(* Logix 5000 AddOnInstructionDefinition export CM1T_DataExchange; software revision 20.00 *)

TYPE CM1T_DriveStatus :
STRUCT
   StatusValue : SINT;   // Indicates status and error type
   StatusValue1 : SINT;   // Additional status values
   In_Position : BOOL;   // Drive is in position and ready to move
   Moving : BOOL;   // Drive is currently moving
   Disabled : BOOL;   // Drive is disabled
   Error : BOOL;   // Drive is in an error state
   MoveComplete : BOOL;   // Move Complete
   NewStartRequired : BOOL;   // New setpoint required
   HomeAchieved : BOOL;   // Home achieved
END_STRUCT
END_TYPE

TYPE CM1T_Controlword :
STRUCT
   Start : BOOL;   // Start a motion or set a new setpoint
   Halt : BOOL;   // Halt the current motion
   Relative_Move : BOOL;   // Execute the position profile as a relative move
   Speed_Control : BOOL;   // Execute the profile as speed control only
   Disable : BOOL;   // Disable the drive (zero torque)
   Reset_Error : BOOL;   // Reset any existing errors with rising edge
   Set_to_Zero : BOOL;   // Set the current position to 0
   Home : BOOL;   // Execute a home search
END_STRUCT
END_TYPE

TYPE CM1T_Axis :
STRUCT
   Input : SINT[36];   // Data coming from the CM1-T
   Output : SINT[28];   // Data going to the CM1-T
   us50Counter : DINT;   // Controller 50us counter
   ModeOfOperation : SINT;   // Type of motion control mode
   ModeOfOperationDisplay : SINT;   // Indicates the active control mode
   Controlword : CM1T_Controlword;   // Controls the drive operation
   DriveStatus : CM1T_DriveStatus;   // Shows status of the drive
   PositionTarget : DINT;   // Final target position for position move
   SpeedTarget : DINT;   // Maximum speed for target move
   TorqueTarget : INT;   // Max torque allowed in 0.1% of peak. Typically 1100
   AccelerationTarget : INT;   // Acceleration for profile move
   DecelerationTarget : INT;   // Deceleration for profile move
   PositionActual : DINT;   // Actual position of the drive
   TargetActual : DINT;   // 1ms position target
   PositionError : DINT;   // Error between the current drive position and the instantaneous target position
   SpeedActual : DINT;   // Actual speed of the drive
   CurrentActual : INT;   // 0.1% of rated current
   OverloadActual : INT;   // 0.1% of overload torque
   DCVoltage : INT;   // DC voltage bus. 0.1V unit
   AnalogIN : INT;   // Value of 10bit analog input
   DigitalIN : SINT;   // Read the digital inputs
   DigitalOUT : SINT;   // Set the digital outputs
   Temperature : SINT;   // Temperature of the drive
   ErrorCode : SINT;   // Indicates error in Ethernet/IP module
   ReadAddress1 : INT;   // Read Address 1
   ReadValue1 : DINT;   // Value read from register
   ReadValueAddress1 : INT;   // Responding register address
   WriteValue1 : DINT;   // Value to write
   WriteAddress1 : INT;   // Write Address 1
END_STRUCT
END_TYPE

ADD_ON_INSTRUCTION CM1T_DataExchange   (* revision 1.2, vendor Myostat Motion Control, ExecutePrescan *)
// CM1T Data Exchange
VAR_IN_OUT
   DriveInput : AB:ETHERNET_MODULE_SINT_36Bytes:I:0; {required}
   DriveOutput : AB:ETHERNET_MODULE_SINT_28Bytes:O:0; {required}
        .DATA[0]   // Copy outputs to drive
   CM1T_Axis : CM1T_Axis; {required}
        .INPUT   // Copy input from drive
        .OUTPUT[0]   // PositionTarget
        .OUTPUT[4]   // SpeedTarget
        .OUTPUT[8]   // TorqueTarget
        .OUTPUT[10]   // AccelerationTarget
        .OUTPUT[12]   // DecelerationTarget
        .OUTPUT[14]   // Controlword
        .OUTPUT[16]   // ModeOfOperation
        .OUTPUT[17]   // WriteData
        .OUTPUT[18]   // Write Address1
        .OUTPUT[20]   // Write Value1
        .OUTPUT[24]   // Read Address1
        .MODEOFOPERATIONDISPLAY   // Mode Display
        .CONTROLWORD.START   // Controlword.Start Off
        .DRIVESTATUS.STATUSVALUE   // Status
        .DRIVESTATUS.IN_POSITION   // In Position
        .DRIVESTATUS.MOVING   // Moving
        .DRIVESTATUS.ERROR   // Error
        .POSITIONACTUAL   // Position
        .POSITIONERROR   // Position Error
        .SPEEDACTUAL   // Speed
        .CURRENTACTUAL   // Current
        .OVERLOADACTUAL   // Torque
        .DCVOLTAGE   // DC Voltage
        .ANALOGIN   // AnalogIN
        .DIGITALIN   // DigitalIN
        .TEMPERATURE   // Temperature
        .ERRORCODE   // ErrorCode
END_VAR
VAR
   storage_InPosition : BOOL; {access None}
   rising_InPosition : BOOL; {access None}
   counter : DINT; {access None}
   old_counter : DINT; {access None}
   new_MessageCount : DINT; {access None}
END_VAR

ROUTINE Logic   (* ladder *)
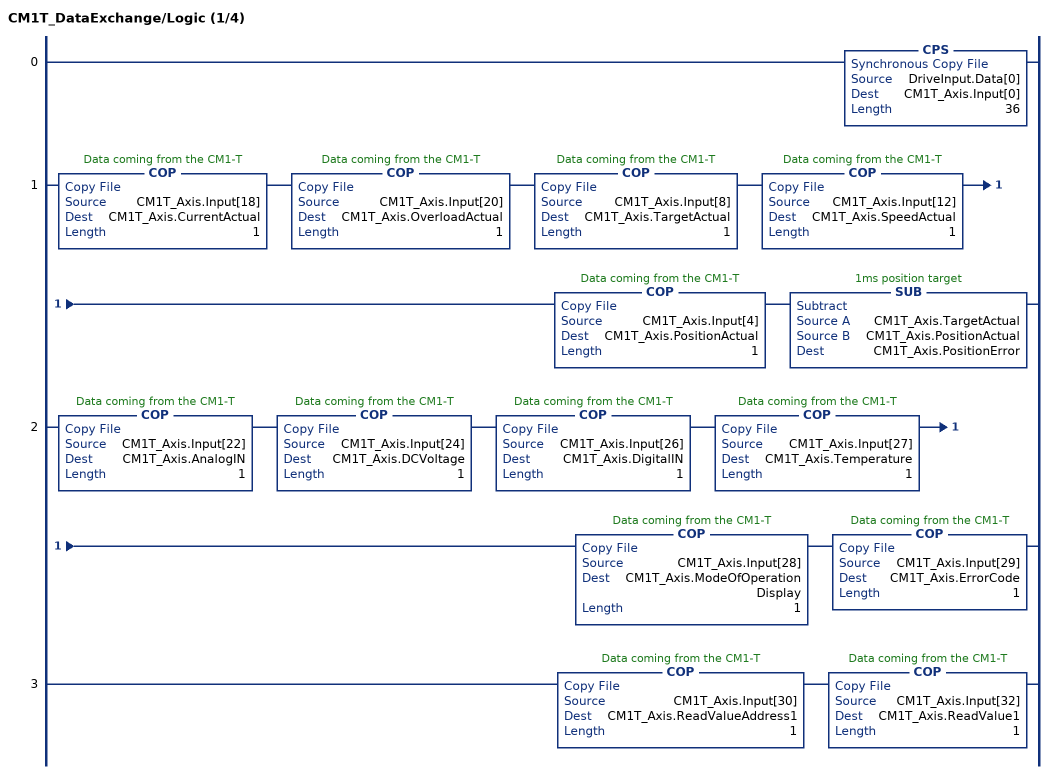
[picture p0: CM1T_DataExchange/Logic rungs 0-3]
   0: CPS(DriveInput.Data[0],CM1T_Axis.Input[0],36);
   1: COP(CM1T_Axis.Input[18],CM1T_Axis.CurrentActual,1)COP(CM1T_Axis.Input[20],CM1T_Axis.OverloadActual,1)COP(CM1T_Axis.Input[8],CM1T_Axis.TargetActual,1)COP(CM1T_Axis.Input[12],CM1T_Axis.SpeedActual,1)COP(CM1T_Axis.Input[4],CM1T_Axis.PositionActual,1)SUB(CM1T_Axis.TargetActual,CM1T_Axis.PositionActual,CM1T_Axis.PositionError);
   2: COP(CM1T_Axis.Input[22],CM1T_Axis.AnalogIN,1)COP(CM1T_Axis.Input[24],CM1T_Axis.DCVoltage,1)COP(CM1T_Axis.Input[26],CM1T_Axis.DigitalIN,1)COP(CM1T_Axis.Input[27],CM1T_Axis.Temperature,1)COP(CM1T_Axis.Input[28],CM1T_Axis.ModeOfOperationDisplay,1)COP(CM1T_Axis.Input[29],CM1T_Axis.ErrorCode,1);
   3: COP(CM1T_Axis.Input[30],CM1T_Axis.ReadValueAddress1,1)COP(CM1T_Axis.Input[32],CM1T_Axis.ReadValue1,1);
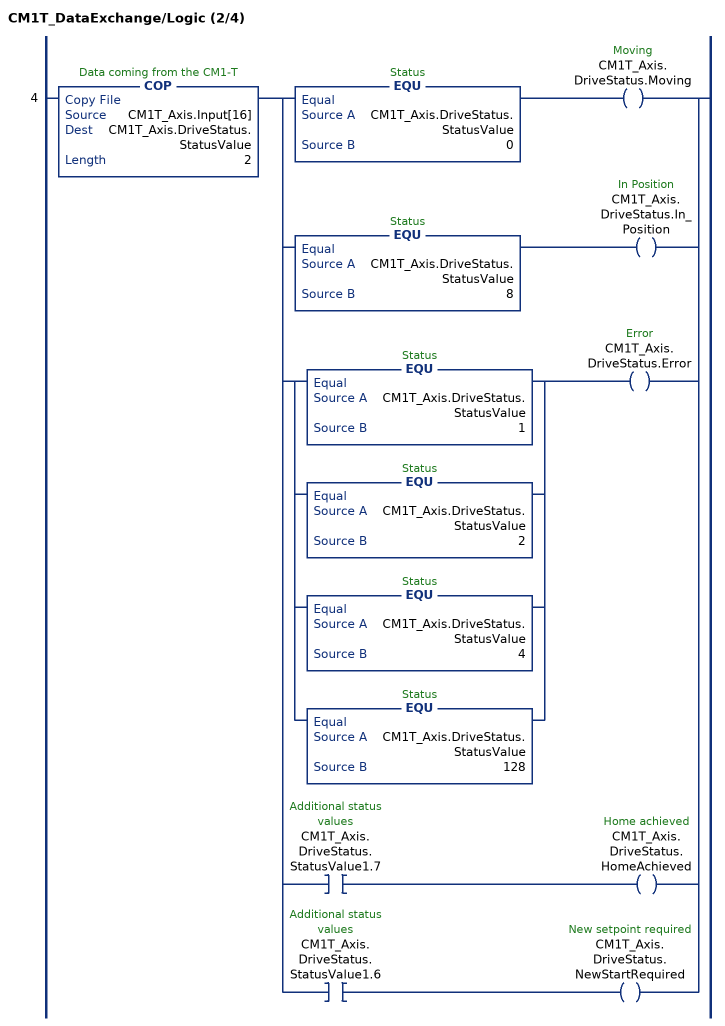
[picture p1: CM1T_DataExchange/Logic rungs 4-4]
   4: COP(CM1T_Axis.Input[16],CM1T_Axis.DriveStatus.StatusValue,2)[EQU(CM1T_Axis.DriveStatus.StatusValue,0) OTE(CM1T_Axis.DriveStatus.Moving) ,EQU(CM1T_Axis.DriveStatus.StatusValue,8) OTE(CM1T_Axis.DriveStatus.In_Position) ,[EQU(CM1T_Axis.DriveStatus.StatusValue,1) ,EQU(CM1T_Axis.DriveStatus.StatusValue,2) ,EQU(CM1T_Axis.DriveStatus.StatusValue,4) ,EQU(CM1T_Axis.DriveStatus.StatusValue,128) ] OTE(CM1T_Axis.DriveStatus.Error) ,XIC(CM1T_Axis.DriveStatus.StatusValue1.7) OTE(CM1T_Axis.DriveStatus.HomeAchieved) ,XIC(CM1T_Axis.DriveStatus.StatusValue1.6) OTE(CM1T_Axis.DriveStatus.NewStartRequired) ];
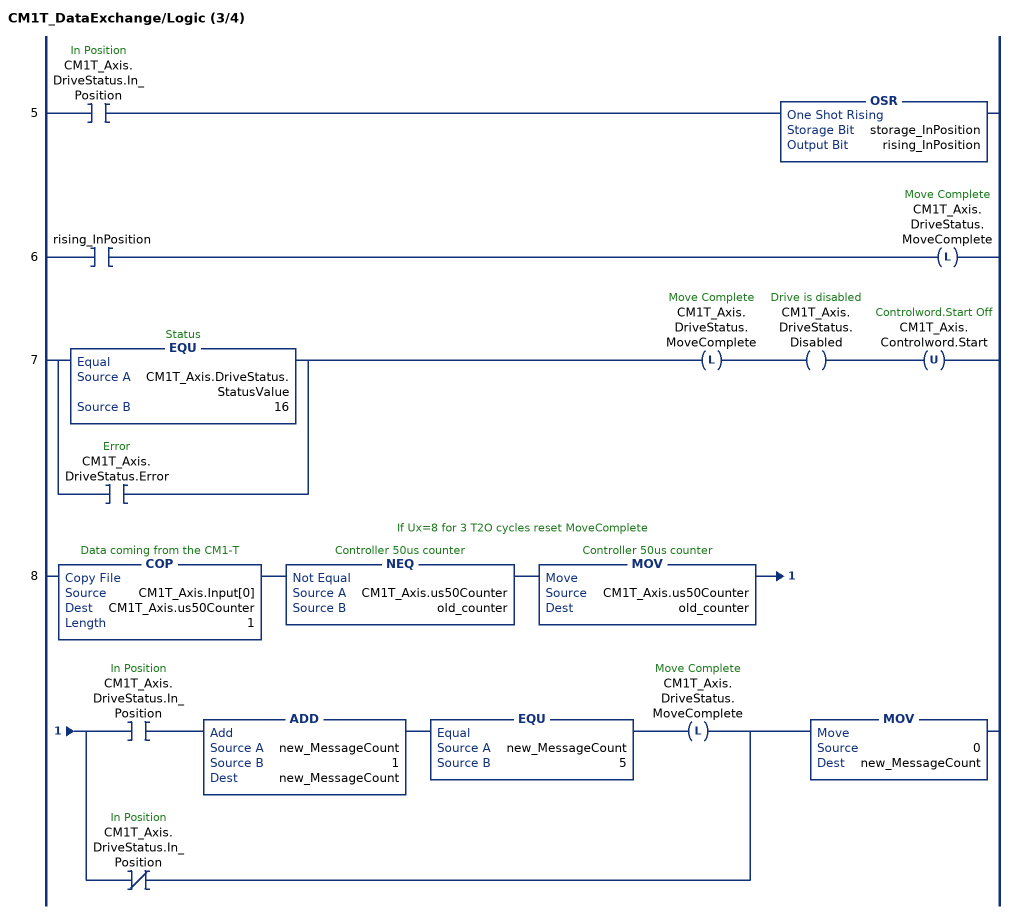
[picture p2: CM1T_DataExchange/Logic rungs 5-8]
   5: XIC(CM1T_Axis.DriveStatus.In_Position)OSR(storage_InPosition,rising_InPosition);
   6: XIC(rising_InPosition)OTL(CM1T_Axis.DriveStatus.MoveComplete);
   7: [EQU(CM1T_Axis.DriveStatus.StatusValue,16) ,XIC(CM1T_Axis.DriveStatus.Error) ]OTL(CM1T_Axis.DriveStatus.MoveComplete)OTE(CM1T_Axis.DriveStatus.Disabled)OTU(CM1T_Axis.Controlword.Start);
   // If Ux=8 for 3 T2O cycles reset MoveComplete
   8: COP(CM1T_Axis.Input[0],CM1T_Axis.us50Counter,1)NEQ(CM1T_Axis.us50Counter,old_counter)MOV(CM1T_Axis.us50Counter,old_counter)[XIC(CM1T_Axis.DriveStatus.In_Position) ADD(new_MessageCount,1,new_MessageCount) EQU(new_MessageCount,5) OTL(CM1T_Axis.DriveStatus.MoveComplete) ,XIO(CM1T_Axis.DriveStatus.In_Position) ]MOV(0,new_MessageCount);
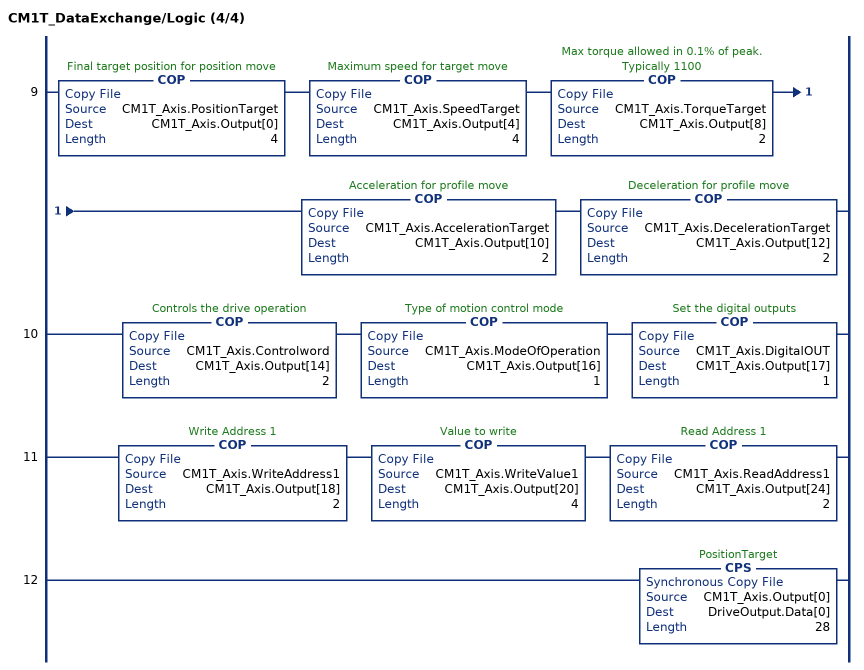
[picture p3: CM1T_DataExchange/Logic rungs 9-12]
   9: COP(CM1T_Axis.PositionTarget,CM1T_Axis.Output[0],4)COP(CM1T_Axis.SpeedTarget,CM1T_Axis.Output[4],4)COP(CM1T_Axis.TorqueTarget,CM1T_Axis.Output[8],2)COP(CM1T_Axis.AccelerationTarget,CM1T_Axis.Output[10],2)COP(CM1T_Axis.DecelerationTarget,CM1T_Axis.Output[12],2);
   10: COP(CM1T_Axis.Controlword,CM1T_Axis.Output[14],2)COP(CM1T_Axis.ModeOfOperation,CM1T_Axis.Output[16],1)COP(CM1T_Axis.DigitalOUT,CM1T_Axis.Output[17],1);
   11: COP(CM1T_Axis.WriteAddress1,CM1T_Axis.Output[18],2)COP(CM1T_Axis.WriteValue1,CM1T_Axis.Output[20],4)COP(CM1T_Axis.ReadAddress1,CM1T_Axis.Output[24],2);
   12: CPS(CM1T_Axis.Output[0],DriveOutput.Data[0],28);
END_ROUTINE

ROUTINE Prescan   (* ladder *)
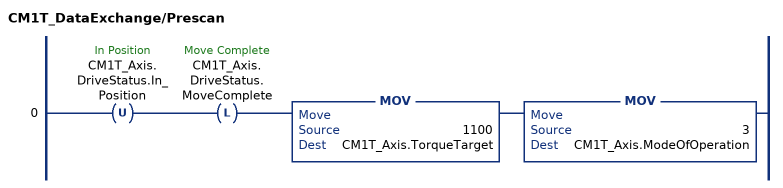
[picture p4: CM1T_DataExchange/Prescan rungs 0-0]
   0: OTU(CM1T_Axis.DriveStatus.In_Position)OTL(CM1T_Axis.DriveStatus.MoveComplete)MOV(1100,CM1T_Axis.TorqueTarget)MOV(3,CM1T_Axis.ModeOfOperation);
END_ROUTINE
END_ADD_ON_INSTRUCTION
